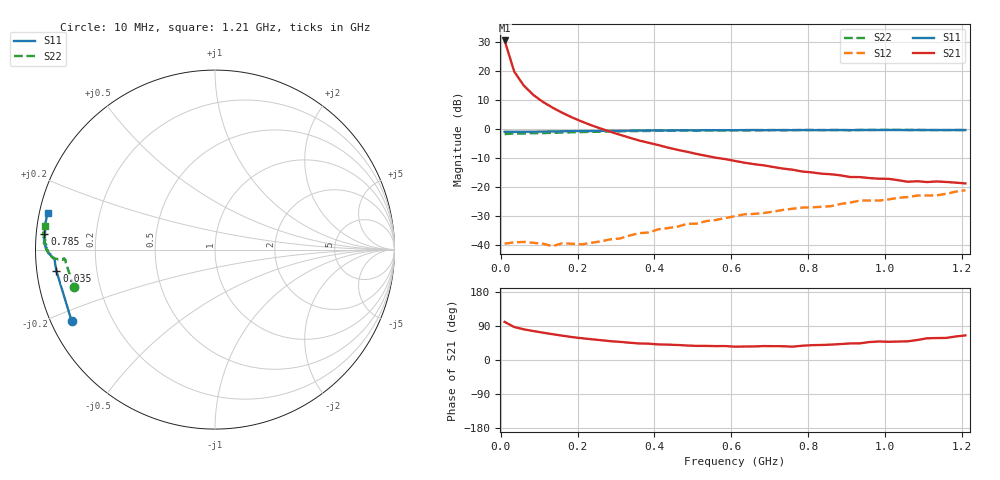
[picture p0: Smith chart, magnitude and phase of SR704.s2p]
!  POLYFET RF DEVICES
!  S PARAMETERS FOR
!  SR704 (EACH SIDE)
!  VDS=28, IDQ=800MA
! S1A4+4Die, AR pkg, left side, Vds=28Vdc, Idq=800ma, Vgsth=2.63Vdc,
! Date: Mon Jul 27 15:55:45 1998
# MHZ  S  MA  R  50.0000
! SCATTERING PARAMETERS :
! Freq=MHz Mag[s11] Ang[s11] Mag[s21] Ang[s21] Mag[s12] Ang[s12] Mag[s22] Ang[s22]
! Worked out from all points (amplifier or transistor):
!   49 points, 10 MHz to 1.21 GHz, reference 50 ohm
!   highest |S21| = 30.4 dB at 10 MHz (marker M1)
!   |S21| within 3 dB of that: start of sweep to 17.01 MHz
!   unconditionally stable (mu >= 1): 141.3 MHz to end of sweep
!   at 210 MHz: K = 1.32, MAG = 17.7 dB, |S12| = -39.7 dB
!   at 610 MHz: K = 1.22, MAG = 6.7 dB, |S12| = -30.0 dB
!   at 1.21 GHz: K = 1.29, MAG = -2.0 dB, |S12| = -21.1 dB
!   S11 on the Smith chart (normalised r, x): 10 MHz: 0.06, -0.23; 35 MHz: 0.06, -0.07; 785 MHz: 0.02, +0.05; 1.21 GHz: 0.02, +0.11
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10  0.8922 -153.6  33 100.5  0.01069 14.6  0.8131 -165.2
35  0.8914 -172.3  9.634 87.0  0.01125 8.0  0.8345 -174.9
60  0.8944 -175.1  5.54 80.9  0.01145 11.4  0.8351 -176.1
85  0.8951 -176.4  3.82 76.4  0.01104 13.6  0.8437 -176.7
110  0.9002 -176.7  2.899 72.1  0.01067 16.3  0.8456 -176.2
135  0.9043 -177.1  2.314 68.1  0.00968 21.4  0.8582 -176.2
160  0.9074 -177.5  1.891 64.3  0.01086 28.4  0.8649 -176.4
185  0.9133 -177.8  1.581 60.6  0.01066 38.9  0.8752 -176.4
210  0.9187 -178.2  1.344 57.6  0.01037 42.0  0.8812 -176.6
235  0.9185 -178.5  1.16 54.9  0.01106 49.5  0.8918 -176.7
285  0.9289 -178.8  0.8936 49.7  0.01266 63.2  0.9033 -177.3
360  0.9371 -179.9  0.632 43.6  0.01617 76.5  0.9173 -178.2
410  0.942 179.5  0.5276 41.1  0.01883 84.1  0.9264 -178.9
510  0.9425 178.2  0.3711 37.2  0.02362 88.8  0.9298 -179.5
610  0.949 177.1  0.2813 35.1  0.03164 96.6  0.9476 178.9
785  0.9542 174.8  0.1853 37.7  0.04444 98.6  0.9548 176.8
810  0.9519 174.6  0.1792 39.1  0.04497 100.0  0.959 176.4
935  0.9587 172.6  0.1489 44.0  0.05876 102.7  0.9553 175.4
1010  0.9575 171.5  0.1388 48.0  0.06147 104.0  0.9618 174.4
1060  0.9558 170.4  0.1236 49.3  0.06761 105.2  0.9568 173.8
1135  0.9555 169.3  0.1251 57.9  0.07219 105.5  0.9517 172.9
1210  0.9551 167.6  0.1158 65.0  0.08842 105.2  0.9539 172.1
